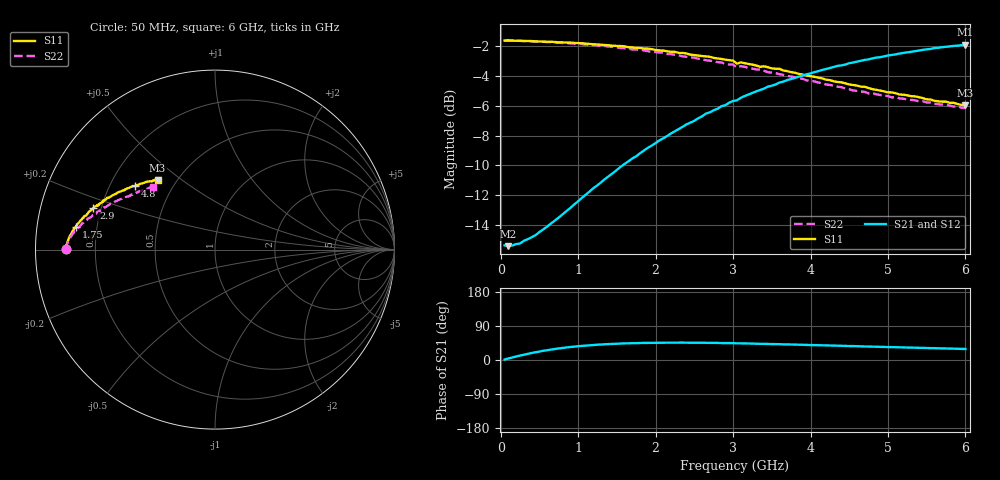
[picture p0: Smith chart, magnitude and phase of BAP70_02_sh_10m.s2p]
!	Created	by	janssen	on	Thu	Dec	12	13:21:33	MET	2002
#	HZ	S	MA	R	50
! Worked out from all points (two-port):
!   120 points, 50 MHz to 6 GHz, reference 50 ohm
!   highest |S21| = -1.90 dB at 6 GHz (marker M1); lowest = -15.4 dB at 100 MHz (marker M2)
!   |S21| within 3 dB of the highest: 3.372 GHz to end of sweep
!   lowest |S11| = -6.0 dB at 6 GHz (marker M3), VSWR 3.03, Z = 19.7 + j20.5 ohm
!   |S11| at or under -10 dB: nowhere
!   |S22| runs from -6.2 to -1.6 dB; largest |S21 - S12| = 0.015
!   S11 on the Smith chart (normalised r, x): 50 MHz: 0.09, +0.00; 1.75 GHz: 0.12, +0.08; 2.9 GHz: 0.17, +0.16; 4.8 GHz: 0.30, +0.32; 6 GHz: 0.39, +0.41
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5e7  0.8298 179.9  0.1703 1.2  0.1693 1.2  0.8306 179.9
1e8  0.8303 179.6  0.1693 4.1  0.1698 3.9  0.8307 179.5
2.5e8  0.8286 178.7  0.1729 11.7  0.1734 11.5  0.8279 178.7
4e8  0.8269 178.0  0.1814 18.5  0.1809 18.2  0.8247 178.0
7.5e8  0.8188 176.3  0.2113 30.5  0.211 30.2  0.8162 176.3
1.05e9  0.8132 174.7  0.2462 37.3  0.2452 37.0  0.8072 174.9
1.75e9  0.7844 170.6  0.3392 44.5  0.3384 44.3  0.774 171.1
2.05e9  0.7692 168.2  0.3838 45.4  0.38 45.4  0.7573 169.3
2.65e9  0.7343 163.5  0.4721 45.4  0.464 45.3  0.7129 165.2
2.9e9  0.7161 161.2  0.5035 44.7  0.498 44.6  0.6921 163.1
3e9  0.711 160.3  0.5203 44.4  0.5141 44.1  0.6895 162.2
3.05e9  0.6941 159.1  0.523 43.9  0.5163 44.1  0.6734 161.7
3.1e9  0.7013 159.4  0.533 43.9  0.5274 44.0  0.6814 161.6
3.35e9  0.6775 156.8  0.5665 42.7  0.5595 42.9  0.6628 159.2
3.6e9  0.667 154.3  0.5999 41.7  0.5891 41.9  0.6399 157.1
4.05e9  0.6271 149.4  0.65 39.2  0.6428 39.7  0.6054 152.9
4.3e9  0.6055 147.0  0.6766 38.0  0.6679 38.3  0.5858 150.2
4.35e9  0.6026 146.0  0.6824 37.8  0.6753 38.3  0.581 150.3
4.8e9  0.5698 141.5  0.7232 35.2  0.7149 35.8  0.5524 145.8
5.05e9  0.5559 138.8  0.7427 33.9  0.7368 34.7  0.5349 143.4
5.55e9  0.5262 133.6  0.7781 31.4  0.7723 32.1  0.514 138.4
6e9  0.5034 129.5  0.804 29.1  0.8047 30.0  0.4918 135.0
